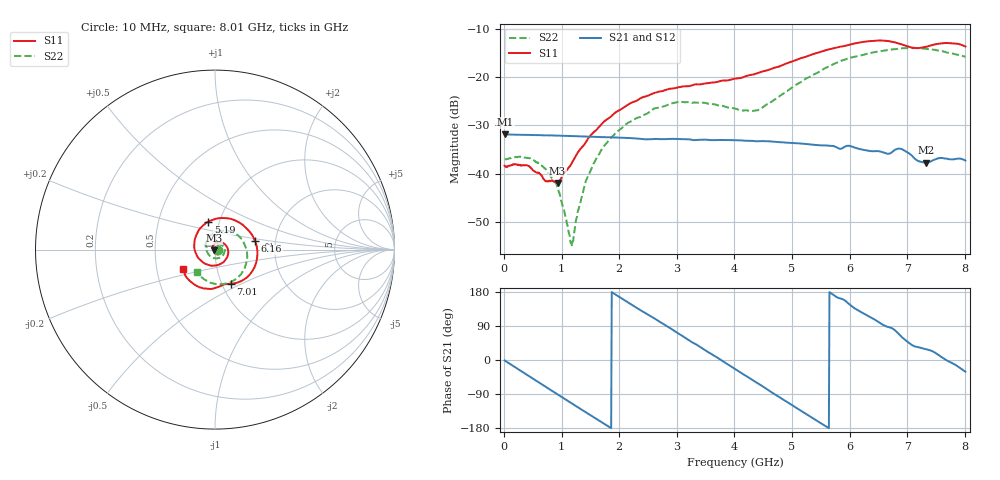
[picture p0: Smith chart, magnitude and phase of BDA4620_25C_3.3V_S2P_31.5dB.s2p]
!Agilent Technologies,E5071B,MY42404982,A.09.10
!Date: Wed May 06 08:55:44 2026
!Data & Calibration Information:
!Freq	S11:SOLT2(ON)	S21:SOLT2(ON)	S12:SOLT2(ON)	S22:SOLT2(ON)
# Hz S RI R 50
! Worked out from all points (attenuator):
!   801 points, 10 MHz to 8.01 GHz, reference 50 ohm
!   highest |S21| = -31.86 dB at 20 MHz (marker M1); lowest = -37.7 dB at 7.33 GHz (marker M2)
!   lowest |S11| = -42.0 dB at 930 MHz (marker M3), VSWR 1.02, Z = 49.4 - j0.493 ohm
!   |S11| at or under -10 dB: start of sweep to end of sweep
!   |S22| runs from -55.1 to -13.9 dB; largest |S21 - S12| = 0.00017
!   S11 on the Smith chart (normalised r, x): 10 MHz: 1.02, -0.00; 5.19 GHz: 0.89, +0.28; 6.16 GHz: 1.57, +0.16; 7.01 GHz: 1.10, -0.44; 8.01 GHz: 0.68, -0.16
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1e7  0.012 -0.000714  0.0255 -0.000522  0.0256 -0.000561  0.014 -0.000467
2e7  0.0118 -0.000645  0.0255 -0.000898  0.0255 -0.00102  0.0141 -0.000326
4.9e8  0.0078 -0.00784  0.0168 -0.0186  0.0168 -0.0187  0.0129 -0.00541
7.2e8  0.000816 -0.00829  0.00838 -0.0235  0.00836 -0.0236  0.0085 -0.00727
9.3e8  -0.00623 -0.00499  -0.000331 -0.0248  -0.000311 -0.0248  0.00362 -0.00625
1.17e9  -0.0119 0.00413  -0.00992 -0.0224  -0.00999 -0.0224  -0.00157 -0.0011
1.35e9  -0.013 0.0134  -0.016 -0.0183  -0.016 -0.0183  -0.00354 0.00449
1.53e9  -0.00986 0.0239  -0.0206 -0.0126  -0.0205 -0.0127  -0.00337 0.0112
1.77e9  0.00117 0.0358  -0.0236 -0.00359  -0.0236 -0.00357  0.000663 0.0204
2.14e9  0.0303 0.0414  -0.0209 0.0106  -0.0209 0.0106  0.0164 0.0289
2.68e9  0.0702 0.00806  -0.00513 0.0222  -0.00513 0.0222  0.044 0.0196
3.08e9  0.0684 -0.0411  0.00966 0.0206  0.00969 0.0207  0.0551 -0.00703
4.01e9  -0.0596 -0.0761  0.0203 -0.00889  0.0203 -0.00891  -0.01 -0.0463
4.43e9  -0.1117 -0.00726  0.0096 -0.0194  0.00959 -0.0195  -0.0444 -0.0118
5.19e9  -0.0373 0.1558  -0.015 -0.0138  -0.0151 -0.0138  -0.0053 0.0917
5.35e9  0.0079 0.1726  -0.0177 -0.00919  -0.0178 -0.0092  0.023 0.1015
6.16e9  0.2241 0.047  -0.0116 0.0138  -0.0116 0.0139  0.1641 0.0298
6.68e9  0.1855 -0.1479  0.000969 0.016  0.00102 0.016  0.1696 -0.0896
7.01e9  0.0867 -0.1901  0.0111 0.0122  0.0112 0.0122  0.122 -0.1598
7.33e9  0.0241 -0.2059  0.0115 0.00612  0.0115 0.00614  0.0455 -0.1922
7.66e9  -0.0856 -0.2101  0.0143 0.000365  0.0143 0.000261  -0.035 -0.1801
8.01e9  -0.1776 -0.11  0.0117 -0.00698  0.0117 -0.007  -0.1012 -0.1274
